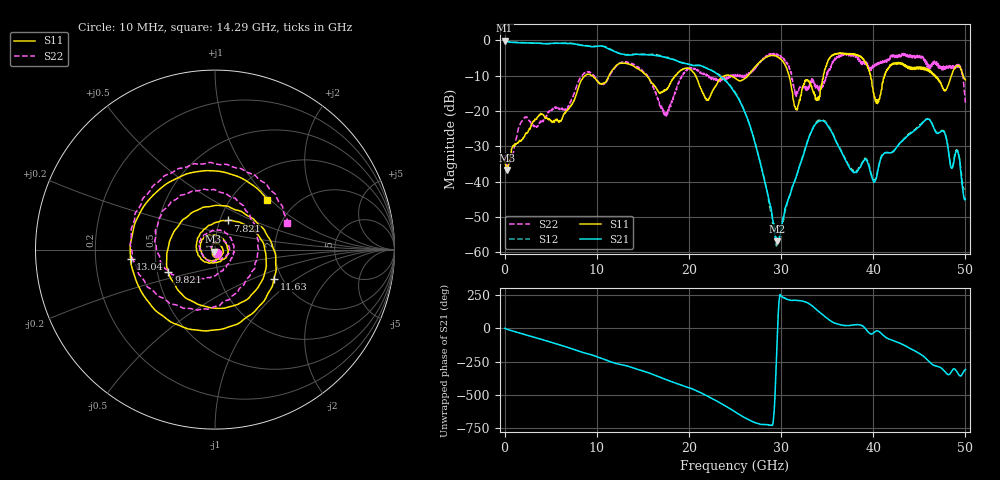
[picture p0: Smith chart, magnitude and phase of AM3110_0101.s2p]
# Hz S DB R 50.0
!freq dBS11 angS11 dBS21 angS21 dBS12 angS12 dBS22 angS22
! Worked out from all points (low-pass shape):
!   1601 points, 10 MHz to 50 GHz, reference 50 ohm
!   highest |S21| = -0.16 dB at 10 MHz (marker M1); lowest = -56.8 dB at 29.54 GHz (marker M2)
!   |S21| within 3 dB of the highest: start of sweep to 11.9 GHz
!   lowest |S11| = -36.7 dB at 259.9 MHz (marker M3), VSWR 1.03, Z = 49.2 - j1.19 ohm
!   |S11| at or under -10 dB: start of sweep to 8.761 GHz; 20.73 GHz to 23.96 GHz (3.23 GHz wide, 14.5 % of centre); 30.87 GHz to 34.59 GHz (3.725 GHz wide, 11.4 % of centre)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
!   |S22| runs from -35.6 to -3.7 dB; largest |S21 - S12| = 0.029
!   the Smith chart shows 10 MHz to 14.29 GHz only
!   S11 on the Smith chart (normalised r, x): 10 MHz: 1.01, -0.04; 7.821 GHz: 1.09, +0.36; 9.821 GHz: 0.57, -0.16; 11.63 GHz: 1.81, -0.67; 13.04 GHz: 0.36, -0.05; 14.29 GHz: 1.45, +0.96
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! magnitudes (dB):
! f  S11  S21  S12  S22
! 10 MHz  -34.3  -0.2  -0.1  -32.5
! 259.9 MHz  -36.7  -0.4  -0.3  -35.3
! 2.01 GHz  -27.8  -0.7  -0.7  -22.4
! 7.821 GHz  -15.1  -1.2  -1.1  -13.1
! 8.352 GHz  -11.2  -1.5  -1.4  -10.1
! 9.821 GHz  -10.8  -1.8  -1.7  -10.4
! 11.63 GHz  -8.7  -2.9  -2.7  -9.0
! 13.04 GHz  -6.5  -4.1  -4.0  -6.0
! 14.29 GHz  -7.9  -4.0  -3.9  -7.4
! 16.69 GHz  -14.5  -4.5  -4.2  -17.1
! 20.07 GHz  -8.1  -6.9  -6.8  -7.8
! 22.01 GHz  -17.0  -8.1  -8.0  -9.7
! 25 GHz  -10.7  -15.0  -14.6  -10.0
! 29.54 GHz  -4.6  -56.8  -58.2  -3.9
! 31.63 GHz  -19.6  -38.7  -38.6  -15.3
! 33.35 GHz  -13.1  -25.6  -25.3  -10.9
! 37.75 GHz  -3.8  -37.1  -36.6  -4.1
! 40.1 GHz  -15.7  -40.1  -39.6  -6.9
! 41.69 GHz  -7.7  -31.8  -31.8  -5.8
! 46.03 GHz  -8.7  -22.3  -22.3  -7.0
! 49.16 GHz  -7.1  -31.5  -31.1  -7.6
! 50 GHz  -11.2  -44.8  -42.1  -17.7
